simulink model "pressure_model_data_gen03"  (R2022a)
settings: Solver=VariableStepAuto  StartTime=0.0  StopTime=tfin  RelTol=1e-3
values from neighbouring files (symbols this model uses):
  Ts = 5    [sisopres.m]

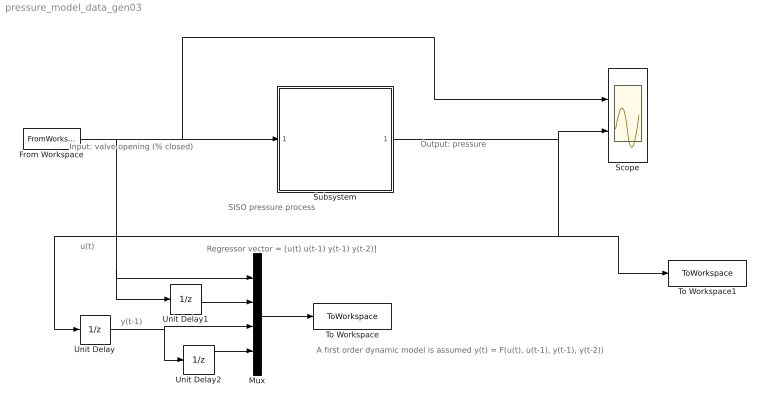
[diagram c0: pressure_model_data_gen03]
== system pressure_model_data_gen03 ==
  note: Regressor vector = [u(t) u(t-1) y(t-1) y(t-2)]
  note: y(t-1)
  note: u(t)
  note: A first order dynamic model is assumed y(t) = F(u(t), u(t-1), y(t-1), y(t-2))
  note: Output: pressure
  note: Input: valve opening (% closed)
  note: SISO pressure process
  From Workspace : FromWorkspace  VariableName=[tsim U]  SampleTime=Ts
  Mux : Mux
  Scope : Scope  NumInputPorts=2
  Subsystem : Subsystem
  To Workspace : ToWorkspace  VariableName=Psim  SampleTime=Ts
  To Workspace1 : ToWorkspace  VariableName=Tsim  SampleTime=Ts
  Unit Delay : UnitDelay  SampleTime=Ts  HasFrameUpgradeWarning=on
  Unit Delay1 : UnitDelay  SampleTime=Ts  HasFrameUpgradeWarning=on
  Unit Delay2 : UnitDelay  SampleTime=Ts  HasFrameUpgradeWarning=on
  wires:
  From Workspace/1 -> Scope/1, Subsystem/1(u), Unit Delay1/1, Mux/1
  Subsystem/1(y) -> Unit Delay/1, To Workspace1/1, Scope/2
  Mux/1 -> To Workspace/1
  Unit Delay1/1 -> Mux/2
  Unit Delay/1 -> Unit Delay2/1, Mux/3
  Unit Delay2/1 -> Mux/4

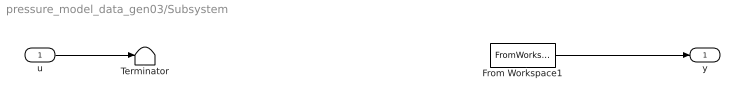
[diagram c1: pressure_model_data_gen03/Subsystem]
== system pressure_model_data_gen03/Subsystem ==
  u : Inport
  From Workspace1 : FromWorkspace  VariableName=[tsim Y]  SampleTime=Ts
  Terminator : Terminator
  y : Outport
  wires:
  From Workspace1/1 -> y/1
  u/1 -> Terminator/1
